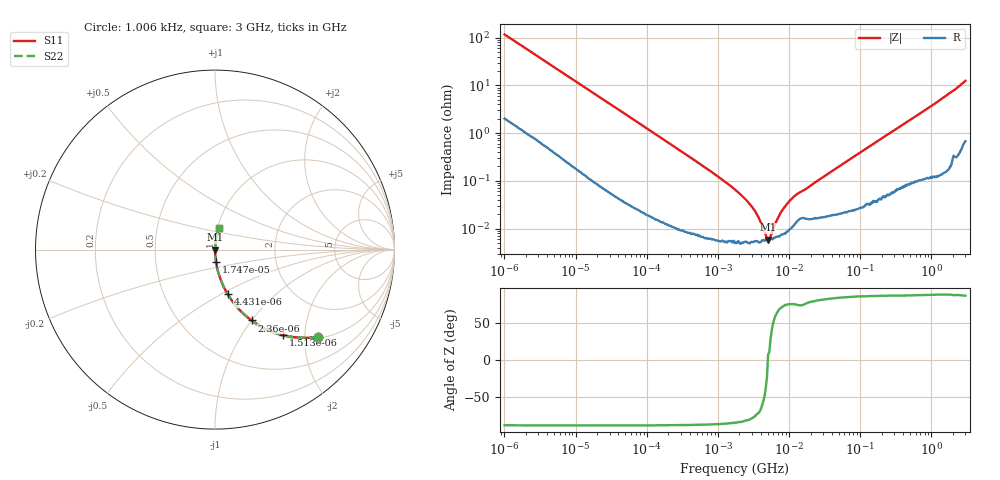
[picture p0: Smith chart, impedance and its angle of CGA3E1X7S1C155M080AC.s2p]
! S-Parameter Data Generated by TDK Corporation
! Copyright(C) 2022 TDK Corporation.
! All Rights Reserved.
! TDK P/N: CGA3E1X7S1C155M080AC (Multilayer Ceramic Chip Capacitor)
! Property: C=1.5uF
! Size(LxWxT): 1.6x0.8x0.8mm
! Model Type: s2p (Touchstone File Format Version 1.0)
! Frequency: DC=Yes Start=0.001006039MHz Stop=3000MHz 479points Log-sweep
! Model Generated on Apr. 15, 2022
! Port Assignments:
!  1 ---| |--- 2
! Applicable Conditions:
!  Temperature = 25 degC
!  DC Bias Voltage = 0 V
!  Small Signal Operation
! Terms and conditions regarding TDK Simulation Models
! (1)This simulation model is being provided solely for informational purposes. Please refer to the specifications of the products in terms of detailed characteristics of such products.
! (2)In no event shall TDK Corporation of any of its subsidiaries be liable for any loss or damage arising, directly or indirectly,
!  From any information contained in this simulation model, including, but not limited to loss or damages arising from any inaccuracies, omissions or errors in connection with such information.
! (3)Any and all copyrights on this simulation model are owned by TDK Corporation.
!  Duplication or redistribution of this simulation model without prior written permission from TDK Corporation is prohibited.
! (4)This simulation model is subject to any modification or change without any prior notice.
! (5)Neither TDK Corporation nor any of its subsidiaries shall make any warranty, express or implied,
!  Including but not limited to the correctness, implied warranties of merchantability and fitness for a particular purpose with respect to this simulation models.
! (6)The use of this simulation model shall be deemed to have consented to the terms and conditions hereof.
# Hz S MA R 50
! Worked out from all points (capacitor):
!   478 points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, 1.006 kHz to 3 GHz, reference 50 ohm
!   read as one part in series: C = 1.36 uF near 1.083 kHz
!   lowest |Z| = 5.87 mohm at 5.073 MHz (marker M1)
!   series resonance near 5.03 MHz, so ESL is about 740 pH
!   S11 on the Smith chart (normalised r, x): 1.006 kHz: 1.04, -2.32; 1.513 kHz: 1.03, -1.55; 2.36 kHz: 1.02, -1.00; 4.431 kHz: 1.01, -0.54; 17.47 kHz: 1.00, -0.14; 3 GHz: 1.01, +0.25
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1006.039  0.7517 -40.3  0.6466 48.7  0.6466 48.7  0.7517 -40.3
1512.504  0.6083 -51.6  0.7833 37.5  0.7833 37.5  0.6083 -51.6
2359.807  0.4445 -62.6  0.8882 26.4  0.8882 26.4  0.4445 -62.6
4431.473  0.2589 -74.1  0.9617 15.0  0.9617 15.0  0.2589 -74.1
12511.27  0.09686 -83.6  0.9939 5.6  0.9939 5.6  0.09686 -83.6
17465.72  0.07003 -85.2  0.9966 4.0  0.9966 4.0  0.07003 -85.2
149930.4  0.008413 -88.5  0.9998 0.5  0.9998 0.5  0.008413 -88.5
794903.8  0.001576 -87.7  0.9999 0.1  0.9999 0.1  0.001576 -87.7
1796709  0.0006302 -85.3  0.9999 0.0  0.9999 0.0  0.0006302 -85.3
2416932  0.0004196 -82.7  0.9999 0.0  0.9999 0.0  0.0004196 -82.7
3132945  0.0002611 -78.5  0.9999 0.0  0.9999 0.0  0.0002611 -78.5
4373588  0.0001012 -55.1  0.9999 0.0  0.9999 0.0  0.0001012 -55.1
4710147  7.248e-05 -37.4  0.9999 0.0  0.9999 0.0  7.248e-05 -37.4
5072606  5.872e-05 7.5  0.9999 -0.0  0.9999 -0.0  5.872e-05 7.5
5669257  7.787e-05 37.7  0.9999 -0.0  0.9999 -0.0  7.787e-05 37.7
6105522  0.0001071 53.3  0.9999 -0.0  0.9999 -0.0  0.0001071 53.3
8213144  0.0002524 72.5  0.9999 -0.0  0.9999 -0.0  0.0002524 72.5
1.104832e7  0.0004318 75.5  0.9999 -0.0  0.9999 -0.0  0.0004318 75.5
2.153109e7  0.0008547 79.2  0.9998 -0.0  0.9998 -0.0  0.0008547 79.2
2.507343e8  0.009667 86.5  0.9995 -0.6  0.9995 -0.6  0.009667 86.5
1.171007e9  0.04341 85.9  0.9978 -2.5  0.9978 -2.5  0.04341 85.9
3e9  0.1224 79.9  0.9858 -7.0  0.9858 -7.0  0.1224 79.9
